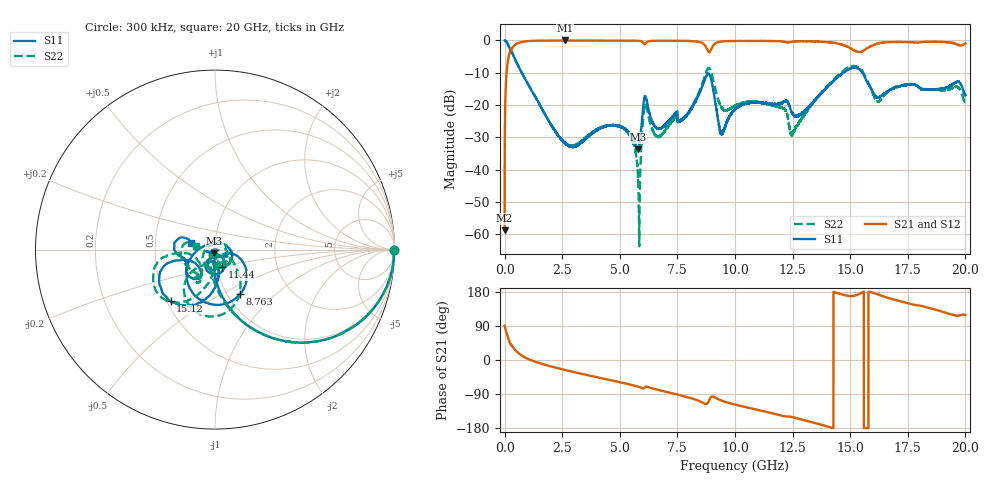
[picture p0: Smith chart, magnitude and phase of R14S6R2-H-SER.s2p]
!{R14S6R2}
!Johanson Technology Inc.
!www.johansontechnology.com
!Test Board Conditions:
!Substrate Type  RO4350B
!Substrate Thickness  20 mil
!Substrate Dk  3.66
!TL Type: GCPW
!TL Trace Width  36 mil
!TL Gap  12 mil
!Electrode orientation  Horizontal
!DUT TOPOLOGY	SERIES
!Mounting Pad LxW  26x36 mil
! Created Wed Nov 25 17:33:21 2020
! 2 Port Network Data from SP1.SP block
! freq  magS11  angS11  magS21  angS21  magS12  angS12  magS22  angS22
# khz S ma R 50
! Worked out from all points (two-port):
!   20001 points, 300 kHz to 20 GHz, reference 50 ohm
!   highest |S21| = -0.01 dB at 2.618 GHz (marker M1); lowest = -58.8 dB at 300 kHz (marker M2)
!   |S21| within 3 dB of the highest: 256 MHz to 8.81 GHz (8.554 GHz wide, 189 % of centre); 8.949 GHz to 15.16 GHz (6.211 GHz wide, 51.5 % of centre)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
!   lowest |S11| = -33.7 dB at 5.787 GHz (marker M3), VSWR 1.04, Z = 49.6 - j2.02 ohm
!   |S11| at or under -10 dB: 740.5 MHz to 14.7 GHz (13.96 GHz wide, 181 % of centre); 14.70394 GHz to 14.70446 GHz (523.8 kHz wide, 0.00356 % of centre); 15.54 GHz to end of sweep
!   |S22| runs from -63.7 to 0.0 dB; largest |S21 - S12| = 0.016
!   S11 on the Smith chart (normalised r, x): 300 kHz: open; 8.763 GHz: 1.15, -0.62; 11.44 GHz: 1.06, -0.21; 15.12 GHz: 0.52, -0.35; 20 GHz: 0.76, +0.06
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300  0.9959 -0.3  0.001153 90.0  0.001177 92.4  0.9951 -0.2
110300  0.9177 -24.4  0.3938 65.5  0.3947 65.4  0.9178 -24.3
283300  0.6645 -50.8  0.7422 38.9  0.7433 38.8  0.6647 -50.7
910300  0.2443 -82.7  0.9678 6.1  0.9669 6.1  0.2457 -84.5
2618300  0.0258 -97.2  0.9985 -26.3  0.998 -26.3  0.02593 -131.6
3334300  0.02641 -139.4  0.9964 -36.4  0.9964 -36.4  0.02754 -110.4
5170300  0.04346 -163.7  0.9947 -60.9  0.9949 -61.0  0.0427 -133.8
5595300  0.02845 -144.3  0.9925 -67.0  0.9923 -67.0  0.02528 -155.3
5787300  0.0206 -99.7  0.9874 -70.1  0.9885 -70.2  0.008527 -174.1
6103300  0.1384 -92.0  0.8823 -71.2  0.8846 -71.2  0.1045 -99.2
6667300  0.04276 -89.2  0.9918 -79.1  0.9907 -79.1  0.03212 112.4
7905300  0.06968 -17.7  0.9841 -97.5  0.9833 -97.5  0.06923 -11.8
8763300  0.2843 -60.6  0.766 -116.0  0.7651 -116.0  0.3307 -72.1
9407300  0.0367 98.7  0.9607 -107.0  0.9622 -106.9  0.09214 -116.2
1.00003e7  0.0856 -0.9  0.98 -117.5  0.9795 -117.6  0.09653 -62.7
1.14363e7  0.1053 -67.8  0.9791 -137.9  0.9795 -137.9  0.103 -30.6
1.24953e7  0.07364 -111.8  0.9599 -150.7  0.9619 -150.7  0.03604 -59.5
1.33343e7  0.1058 -79.9  0.9697 -164.2  0.9713 -164.1  0.1019 -87.7
1.51213e7  0.3796 -130.7  0.7157 168.8  0.7176 168.3  0.4 -140.7
1.61633e7  0.133 -142.0  0.8907 174.1  0.8904 174.0  0.1142 -150.2
1.66673e7  0.1643 -118.7  0.9406 163.5  0.937 163.3  0.1647 -116.8
2e7  0.1396 165.1  0.8955 119.2  0.8942 119.3  0.1071 169.4
